(* Logix 5000 AddOnInstructionDefinition export Bronkhorst_Basic_INT_Input; software revision 37.00 *)

ADD_ON_INSTRUCTION Bronkhorst_Basic_INT_Input   (* revision 1.0, vendor Bronkhorst High-Tech B.V. *)
// Extract data from the Basic INT input connection (in to controller from device)
VAR_IN_OUT
   DataIn : SINT[3]; {required}
END_VAR
VAR_OUTPUT
   Status : SINT; {visible}
   Measure : INT; {visible}
END_VAR

ROUTINE Logic   (* structured text *)
   Status := DataIn[0];
   COP(DataIn[1], Measure, 1);
END_ROUTINE
END_ADD_ON_INSTRUCTION

ADD_ON_INSTRUCTION Bronkhorst_Basic_INT_Output   (* revision 1.0, vendor Bronkhorst High-Tech B.V. *)
// Fill data for the Basic INT output connection (out from controller to device)
VAR_IN_OUT
   DataOut : SINT[2]; {required}   // SINT device output data array
END_VAR
VAR_INPUT
   Setpoint : INT; {visible}   // INT Setpoint
END_VAR

ROUTINE Logic   (* structured text *)
   COP(Setpoint, DataOut[0], 2);
END_ROUTINE
END_ADD_ON_INSTRUCTION
